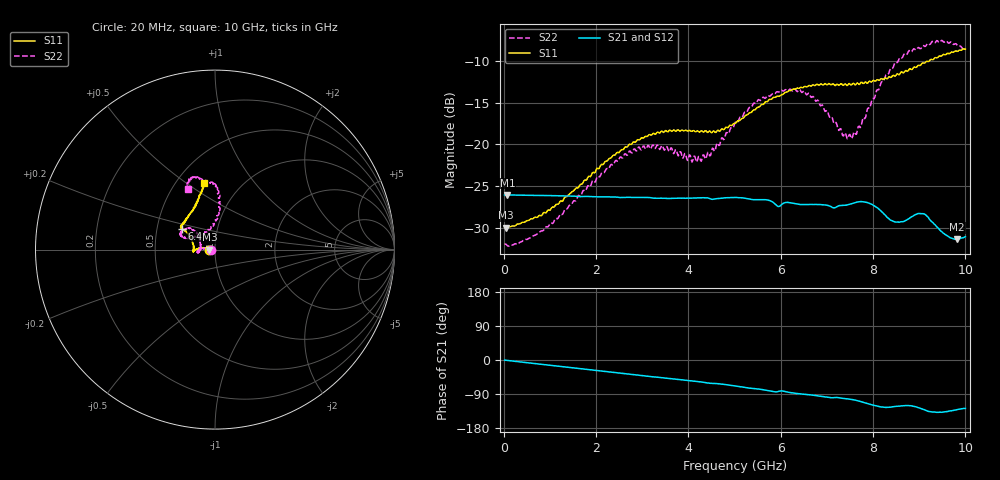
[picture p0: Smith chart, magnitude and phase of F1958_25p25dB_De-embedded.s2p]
! Integrated Device Technology
! Corporate Headquarters
! 6024 Silver Creek Valley Road
! San Jose, CA 95138  USA
! Phone:  1-408-284-8200
! Toll Free:  1-800-223-1366
! Webpage:  http://www.idt.com/
! Timing and RF Division
! 515 Groton Road, Suite 102
! Westford, MA 01886-6024
! Device:  F1958
! Description: 7-bit 0.25 dB Digital Step Attenuator
! Frequency:  0.001 -  6.000 GHz
! Package:  4x4 mm Thin QFN Plastic Package: 24 pin
! Ports:  2 RF, 12 DC
!  Pin  1  = D0
!  Pin  2  = VDD
!  Pin  3  = VMODE
!  Pin  4  = GND
!  Pin  5  = RF1  =  Port 1
!  Pin  6  = GND
!  Pin  7  = GND
!  Pin  8  = GND
!  Pin  9  = GND
!  Pin 10  = GND
!  Pin 11  = GND
!  Pin 12  = GND
!  Pin 13  = GND
!  Pin 14  = RF2  =  Port 2
!  Pin 15  = GND
!  Pin 16  = LE
!  Pin 17  = CLK
!  Pin 18  = DATA
!  Pin 19  = D6
!  Pin 20  = D5
!  Pin 21  = D4
!  Pin 22  = D3
!  Pin 23  = D2
!  Pin 24  = D1
! State:  101
! Atten State:  25.25 dB
! Voltage:  +3.30 Volts
! Current:  0.258 mA
! Data:  The device was measured on a F1958 evaluation board which has
!  individual transmission lines to the RF pins.  Data was collected
!  using a calibrated network analyzer.  The evaluation board was
!  de-embedded using Automatic Fixture Removal (AFR).
!  The reference plane is the edge of the package pin.
! Misc:
!  Action Tracker AT0419
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# GHz S dB R 50
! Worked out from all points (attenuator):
!   500 points, 20 MHz to 10 GHz, reference 50 ohm
!   highest |S21| = -26.07 dB at 80 MHz (marker M1); lowest = -31.4 dB at 9.82 GHz (marker M2)
!   lowest |S11| = -30.0 dB at 40 MHz (marker M3), VSWR 1.07, Z = 46.9 - j0.0428 ohm
!   |S11| at or under -10 dB: start of sweep to 9.157 GHz; 9.180121 GHz to 9.20093 GHz (20.81 MHz wide, 0.226 % of centre)
!   |S22| runs from -32.2 to -7.5 dB; largest |S21 - S12| = 0.00026
!   S11 on the Smith chart (normalised r, x): 20 MHz: 0.94, -0.00; 6.4 GHz: 0.67, +0.17; 10 GHz: 0.68, +0.58
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0.02  -30.00 -178.9  -26.08 -0.3  -26.08 -0.3  -32.03 -178.9
0.04  -30.03 -179.2  -26.08 -0.6  -26.08 -0.5  -31.99 -178.4
0.08  -29.95 179.4  -26.07 -1.1  -26.07 -1.1  -32.19 -178.8
0.84  -28.42 170.9  -26.14 -11.7  -26.13 -11.7  -30.40 172.6
1.7  -24.76 170.7  -26.27 -23.2  -26.26 -23.2  -25.80 171.6
2.62  -20.37 176.8  -26.38 -35.5  -26.35 -35.6  -21.13 -179.4
3.36  -18.60 -176.0  -26.48 -45.8  -26.48 -46.0  -20.40 -169.5
4.24  -18.52 -179.4  -26.43 -57.5  -26.44 -57.5  -21.48 168.8
4.5  -18.58 174.7  -26.59 -61.6  -26.60 -61.7  -20.85 151.5
5.02  -17.45 160.4  -26.38 -68.7  -26.39 -68.6  -17.31 138.3
5.58  -15.20 150.2  -26.65 -77.7  -26.66 -77.6  -14.60 139.9
6.4  -13.23 147.5  -27.20 -89.0  -27.22 -88.9  -13.38 155.6
6.68  -12.87 146.4  -27.22 -92.4  -27.24 -92.3  -14.29 157.5
7.5  -12.71 138.0  -27.20 -103.4  -27.21 -103.3  -18.79 119.7
7.68  -12.68 135.1  -26.91 -107.8  -26.91 -107.8  -17.85 99.9
7.9  -12.48 128.7  -27.04 -115.7  -27.02 -115.8  -15.59 89.6
8.34  -11.87 118.8  -28.92 -124.8  -28.93 -124.8  -11.43 84.0
8.66  -11.38 113.0  -29.29 -120.5  -29.28 -120.8  -9.23 87.7
9.1  -10.20 107.0  -28.35 -130.8  -28.38 -130.7  -8.10 100.2
9.58  -9.16 100.9  -30.90 -136.3  -30.97 -136.6  -7.52 109.1
9.82  -8.79 100.4  -31.44 -131.0  -31.45 -131.0  -8.02 113.1
10  -8.53 99.8  -31.10 -127.8  -31.10 -127.8  -8.63 113.6
